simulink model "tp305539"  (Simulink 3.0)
settings: Solver=ode45  StartTime=0.0  StopTime=5  RelTol=1e-3
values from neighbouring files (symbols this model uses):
  G1den = [0.05 15.008 2.4]    [sl05.m]
  G1num = 0.625    [sl05.m]
  G2den = [6.25 1]    [sl05.m]
  G2num = 12.5    [sl05.m]
undefined symbols (not defined in the file or in its folder): Rden, Rnum
libraries: simulink3 x2

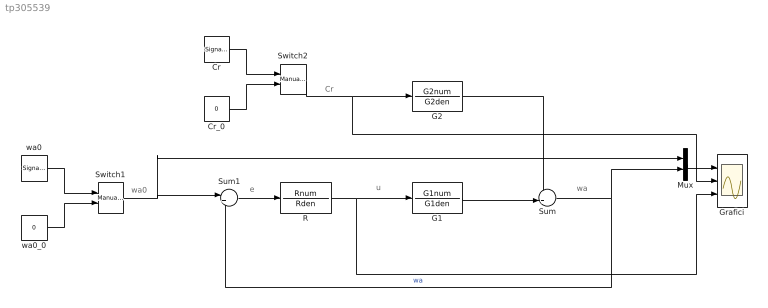
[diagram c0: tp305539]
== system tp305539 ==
  note: u
  note: wa
  note: wa0
  note: Cr
  note: e
  Cr : SignalGenerator  WaveForm=sine  Amplitude=1  Frequency=5  Units=rad/sec
  Cr_0 : Constant  Value=0
  G1 : TransferFcn  Numerator=G1num  Denominator=G1den
  G2 : TransferFcn  Numerator=G2num  Denominator=G2den
  Grafici : Scope  NumInputPorts=3
  Mux : Mux  Inputs=2
  R : TransferFcn  Numerator=Rnum  Denominator=Rden
  Sum : Sum  Inputs=++|  SaturateOnIntegerOverflow=on
  Sum1 : Sum  Inputs=|+-  SaturateOnIntegerOverflow=on
  Switch1 : simulink3/Nonlinear/Manual Switch  sw=1  action=0
  Switch2 : simulink3/Nonlinear/Manual Switch  sw=0  action=0
  wa0 : SignalGenerator  WaveForm=sine  Amplitude=1  Frequency=10  Units=rad/sec
  wa0_0 : Constant  Value=0
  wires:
  R/1 -> G1/1, Grafici/3
  Mux/1 -> Grafici/1
  Sum/1 -> Sum1/2, Mux/2  "wa"
  wa0_0/1 -> Switch1/2
  wa0/1 -> Switch1/1
  Sum1/1 -> R/1
  Switch1/1 -> Sum1/1, Mux/1
  Cr/1 -> Switch2/1
  Cr_0/1 -> Switch2/2
  Switch2/1 -> G2/1, Grafici/2
  G1/1 -> Sum/2
  G2/1 -> Sum/1
